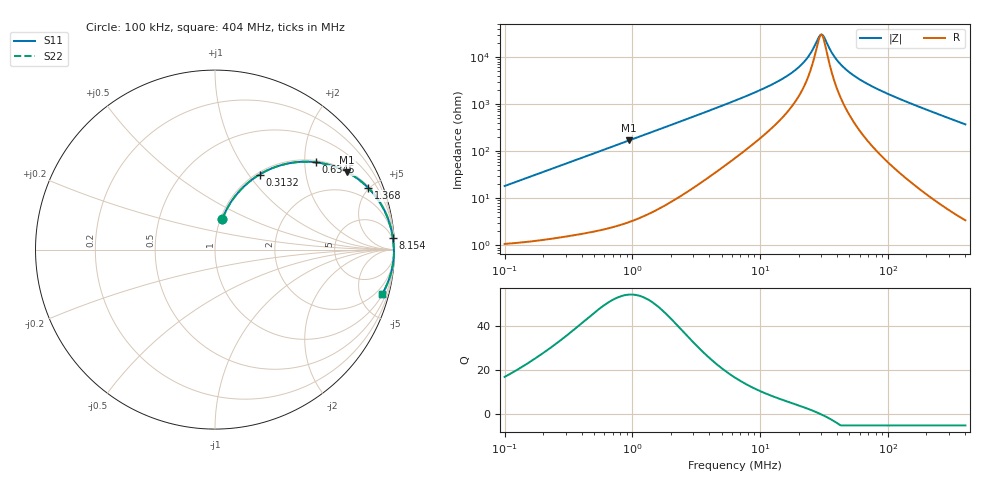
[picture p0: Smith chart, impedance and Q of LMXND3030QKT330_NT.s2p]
! LMXND3030QKT330_NT  S-PARAMETER MODEL  ( Standard Model )
! Model Generated by TAIYO YUDEN Corporation (https://www.yuden.co.jp/en/)
! Version 1.0
! TAIYO YUDEN Control No. 20250925
! Copyright(c) 2025 TAIYO YUDEN CO.,LTD. All Rights Reserved.
! Product Description (link to TY-COMPAS)
! https://ds.yuden.co.jp/TYCOMPAS/or/detail?pn=LMXND3030QKT330MNT&u=M
! Products Name : Inductors
! Characteristics :
!  Inductance : 33 [uH] , SRF(min) : 18 [MHz] , DC Resistance(max) : 0.936 [Ohm]
!  Rated Current : Saturation  400 [mA] , Temp Rise  620 [mA] (40 [degC])
!  Case Size : 3.0 x 3.0 / 0.118 x 0.118 [mm/inch] , Thickness : 1.5 / 0.059 [mm/inch]
!  (Conditions: Temperature = 25 [degC] , DC Bias Current = 0 [A])
! External Node Assignments :
!  1  o---GGG---o  2
! GND o---------o GND
! Frequency Range : 0.1MHz  -  403.964729MHz  [ 402 STEP ]
# MHz S RI R 50
! Freq[MHz].  S11 Real  S11 Imag  S21 Real  S21 Imag  S12 Real  S12 Imag  S22 Real  S22 Imag
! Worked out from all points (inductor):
!   401 points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, 100 kHz to 404 MHz, reference 50 ohm
!   read as one part in series: L = 28.9 uH near 104.2 kHz
!   highest Q = 54.1 at 941.3 kHz (marker M1), where L = 28.6 uH
!   self-resonance near 29.54 MHz
!   S11 on the Smith chart (normalised r, x): 100 kHz: 1.02, +0.36; 313.2 kHz: 1.03, +1.13; 634.5 kHz: 1.05, +2.28; 1.368 MHz: 1.10, +4.91; 8.154 MHz: 3, +31; 404 MHz: 1.07, -7.43
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0.1  0.0417 0.1726  0.9583 -0.1726  0.9583 -0.1726  0.0417 0.1726
0.186413  0.1114 0.2963  0.8886 -0.2963  0.8886 -0.2963  0.1114 0.2963
0.313236  0.2481 0.4182  0.7519 -0.4182  0.7519 -0.4182  0.2481 0.4182
0.401849  0.3472 0.4641  0.6528 -0.4641  0.6528 -0.4641  0.3472 0.4641
0.63447  0.5638 0.4861  0.4362 -0.4861  0.4362 -0.4861  0.5638 0.4861
0.941267  0.7367 0.4313  0.2633 -0.4313  0.2633 -0.4313  0.7367 0.4313
1.367723  0.853 0.3445  0.147 -0.3445  0.147 -0.3445  0.853 0.3445
1.614823  0.8888 0.3042  0.1112 -0.3042  0.1112 -0.3042  0.8888 0.3042
2.828481  0.958 0.1865  0.042 -0.1865  0.042 -0.1865  0.958 0.1865
6.355822  0.988 0.0829  0.012 -0.0829  0.012 -0.0829  0.988 0.0829
8.153837  0.9911 0.063  0.0089 -0.063  0.0089 -0.063  0.9911 0.063
12.60942  0.9941 0.0367  0.0059 -0.0367  0.0059 -0.0367  0.9941 0.0367
17.21603  0.9953 0.0222  0.00467 -0.0222  0.00467 -0.0222  0.9953 0.0222
21.63253  0.996 0.0128  0.00401 -0.0128  0.00401 -0.0128  0.996 0.0128
25.54079  0.9964 0.0063  0.00362 -0.0063  0.00362 -0.0063  0.9964 0.0063
28.92873  0.9966 0.0015  0.00338 -0.0015  0.00338 -0.0015  0.9966 0.0015
30.78768  0.9967 -0.000904  0.00328 0.000904  0.00328 0.000904  0.9967 -0.000904
37.89096  0.997 -0.00909  0.00305 0.00909  0.00305 0.00909  0.997 -0.00909
46.63309  0.997 -0.0178  0.00301 0.0178  0.00301 0.0178  0.997 -0.0178
63.66959  0.9966 -0.0326  0.00345 0.0326  0.00345 0.0326  0.9966 -0.0326
102.6353  0.994 -0.0621  0.006 0.0621  0.006 0.0621  0.994 -0.0621
403.9647  0.9304 -0.2499  0.0696 0.2499  0.0696 0.2499  0.9304 -0.2499
